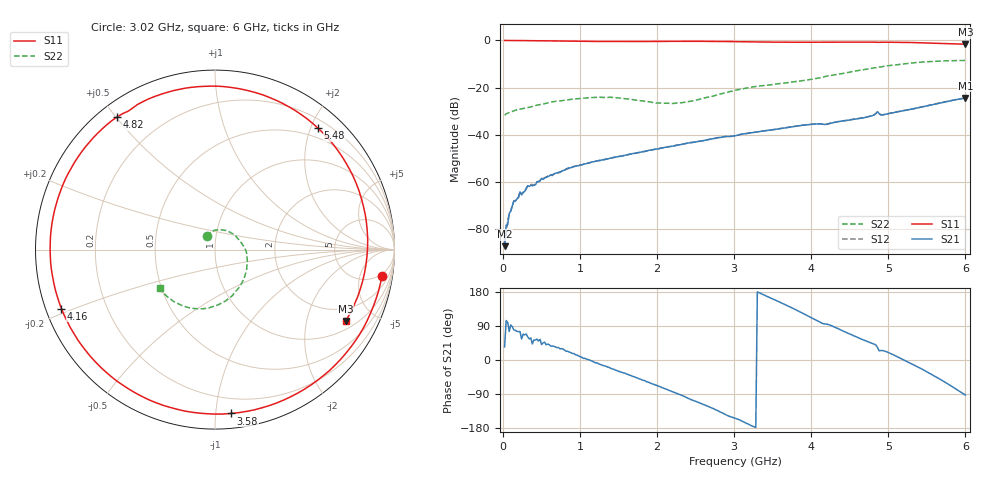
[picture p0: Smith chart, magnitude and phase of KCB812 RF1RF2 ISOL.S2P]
!Agilent Technologies,E5071B,JP1KK00126,A.08.11
!Date: Tue May 14 08:32:55 2013
!Data & Calibration Information:
!Freq	S11:SOLT2(ON)	S21:SOLT2(ON)	S12:SOLT2(ON)	S22:SOLT2(ON)
# Hz S dB R 50
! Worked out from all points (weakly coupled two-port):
!   300 points, 20 MHz to 6 GHz, reference 50 ohm
!   highest |S21| = -24.42 dB at 6 GHz (marker M1); lowest = -87.1 dB at 20 MHz (marker M2)
!   lowest |S11| = -1.6 dB at 6 GHz (marker M3), VSWR 10.77, Z = 67.1 - j172 ohm
!   |S11| at or under -10 dB: nowhere
!   |S22| runs from -31.7 to -8.5 dB; largest |S21 - S12| = 0.0004
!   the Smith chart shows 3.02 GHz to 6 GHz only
!   S11 on the Smith chart (normalised r, x): 3.02 GHz: 4, -11; 3.58 GHz: 0.10, -1.10; 4.16 GHz: 0.04, -0.19; 4.82 GHz: 0.05, +0.50; 5.48 GHz: 0.33, +2.12; 6 GHz: 1.34, -3.43
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2e7  -0.03 -2.5  -87.15 34.7  -86.12 112.3  -31.67 173.9
1.4e8  -0.06 -18.2  -67.97 79.5  -68.14 83.3  -29.79 143.5
2.2e8  -0.07 -28.5  -64.16 75.1  -64.01 74.6  -29.08 130.5
6.2e8  -0.21 -79.7  -56.88 36.5  -56.95 35.0  -26.11 71.3
1.02e9  -0.39 -129.2  -52.65 7.5  -52.69 7.2  -24.56 28.5
1.26e9  -0.46 -158.0  -50.80 -11.6  -50.88 -10.7  -24.10 5.1
1.5e9  -0.48 173.6  -49.19 -30.3  -49.19 -29.4  -24.35 -19.0
2.02e9  -0.43 113.5  -45.90 -69.3  -45.87 -69.3  -26.52 -88.3
2.26e9  -0.39 85.6  -44.41 -88.5  -44.36 -88.6  -26.50 -129.2
2.48e9  -0.39 59.3  -43.09 -107.5  -43.06 -107.7  -25.52 -166.2
2.76e9  -0.43 24.6  -41.46 -131.6  -41.41 -131.3  -23.24 153.1
3.02e9  -0.52 -9.1  -40.34 -154.4  -40.30 -154.3  -21.08 122.4
3.34e9  -0.67 -52.0  -38.53 176.0  -38.51 176.3  -19.26 88.2
3.58e9  -0.75 -84.4  -37.45 153.8  -37.41 153.8  -18.30 62.1
4.02e9  -0.78 -141.9  -35.50 110.0  -35.45 109.9  -16.39 14.3
4.16e9  -0.76 -159.0  -35.56 95.6  -35.52 95.5  -15.51 0.8
4.46e9  -0.72 166.3  -33.91 72.2  -33.80 72.3  -13.65 -32.0
4.82e9  -0.74 126.4  -31.45 41.4  -31.39 41.6  -11.64 -64.4
5.02e9  -0.77 104.7  -30.90 17.9  -30.85 18.1  -10.64 -79.5
5.48e9  -1.04 49.7  -27.90 -28.9  -27.84 -28.6  -9.07 -111.6
5.76e9  -1.34 10.0  -25.89 -61.5  -25.83 -61.4  -8.64 -129.7
6e9  -1.62 -28.6  -24.42 -92.5  -24.36 -92.4  -8.50 -145.1
